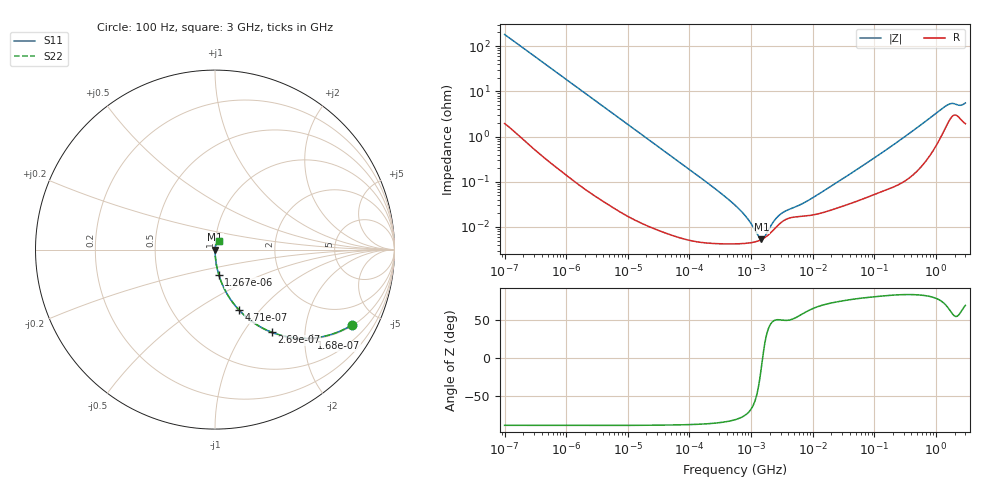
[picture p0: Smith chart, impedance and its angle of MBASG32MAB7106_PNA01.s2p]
! MBASG32MAB7106_PNA01  S-PARAMETER MODEL  ( Standard Model )
! Model Generated by TAIYO YUDEN Corporation (https://www.yuden.co.jp/en/)
! Version 2.0
! TAIYO YUDEN Control No. 250312
! Copyright(c) 2015 TAIYO YUDEN CO.,LTD. All Rights Reserved.
! Product Description (link to TY-COMPAS)
! https://ds.yuden.co.jp/TYCOMPAS/or/detail?pn=MBASG32MAB7106KPNA01&u=M
! Products Name : Multilayer Ceramic Capacitors
! Characteristics :
!  Capacitance : 10 [uF] , Rated Voltage : 35 [V] , TCC : X7R
!  Case Size : 3.2 x 2.5 / 0.126 x 0.098 [mm/inch] , Thickness : 2.5 / 0.098 [mm/inch]
!  (Conditions: Temperature = 25 [degC] , DC Bias Voltage = 0 [V])
! External Node Assignments :
!  1  o---| |---o  2
! GND o---------o GND
! Frequency Range : 100Hz  -  3GHz  [ 401 STEP ]
# MHZ S RI R 50
! Freq[MHz].  S11 Real  S11 Imag  S21 Real  S21 Imag  S12 Real  S12 Imag  S22 Real  S22 Imag
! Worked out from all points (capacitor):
!   401 points, 100 Hz to 3 GHz, reference 50 ohm
!   read as one part in series: C = 8.79 uF near 109 Hz
!   lowest |Z| = 5.37 mohm at 1.474 MHz (marker M1)
!   series resonance near 1.537 MHz, so ESL is about 1.2 nH
!   S11 on the Smith chart (normalised r, x): 100 Hz: 1.04, -3.61; 168 Hz: 1.02, -2.16; 269 Hz: 1.01, -1.35; 471 Hz: 1.01, -0.77; 1.267 kHz: 1.00, -0.29; 3 GHz: 1.04, +0.10
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0.0001  0.763 -0.4199  0.237 0.4199  0.237 0.4199  0.763 -0.4199
0.000168  0.5389 -0.4936  0.4611 0.4936  0.4611 0.4936  0.5389 -0.4936
0.000269  0.3151 -0.4601  0.6849 0.4601  0.6849 0.4601  0.3151 -0.4601
0.000471  0.1324 -0.3349  0.8676 0.3349  0.8676 0.3349  0.1324 -0.3349
0.000724  0.0615 -0.2363  0.9385 0.2363  0.9385 0.2363  0.0615 -0.2363
0.001267  0.0215 -0.1413  0.9785 0.1413  0.9785 0.1413  0.0215 -0.1413
0.001788  0.0112 -0.1014  0.9888 0.1014  0.9888 0.1014  0.0112 -0.1014
0.005476  0.00141 -0.0336  0.9986 0.0336  0.9986 0.0336  0.00141 -0.0336
0.031977  0.000117 -0.00581  0.9999 0.00581  0.9999 0.00581  0.000117 -0.00581
0.231582  4.39e-05 -0.000791  1 0.000791  1 0.000791  4.39e-05 -0.000791
0.547723  4.23e-05 -0.000301  1 0.000301  1 0.000301  4.23e-05 -0.000301
0.740304  4.3e-05 -0.000197  1 0.000197  1 0.000197  4.3e-05 -0.000197
1.09055  4.59e-05 -8.71e-05  1 8.71e-05  1 8.71e-05  4.59e-05 -8.71e-05
1.473992  5.27e-05 -1.05e-05  0.9999 1.05e-05  0.9999 1.05e-05  5.27e-05 -1.05e-05
1.992254  7.04e-05 6.44e-05  0.9999 -6.44e-05  0.9999 -6.44e-05  7.04e-05 6.44e-05
3.198641  0.000131 0.000157  0.9999 -0.000157  0.9999 -0.000157  0.000131 0.000157
9.794414  0.000183 0.000394  0.9998 -0.000394  0.9998 -0.000394  0.000183 0.000394
175.1444  0.00073 0.00563  0.9993 -0.00563  0.9993 -0.00563  0.00073 0.00563
1443.257  0.0177 0.0431  0.9823 -0.0431  0.9823 -0.0431  0.0177 0.0431
1789.813  0.0282 0.0441  0.9718 -0.0441  0.9718 -0.0441  0.0282 0.0441
2419.119  0.0265 0.0397  0.9735 -0.0397  0.9735 -0.0397  0.0265 0.0397
3000  0.0214 0.0497  0.9786 -0.0497  0.9786 -0.0497  0.0214 0.0497
